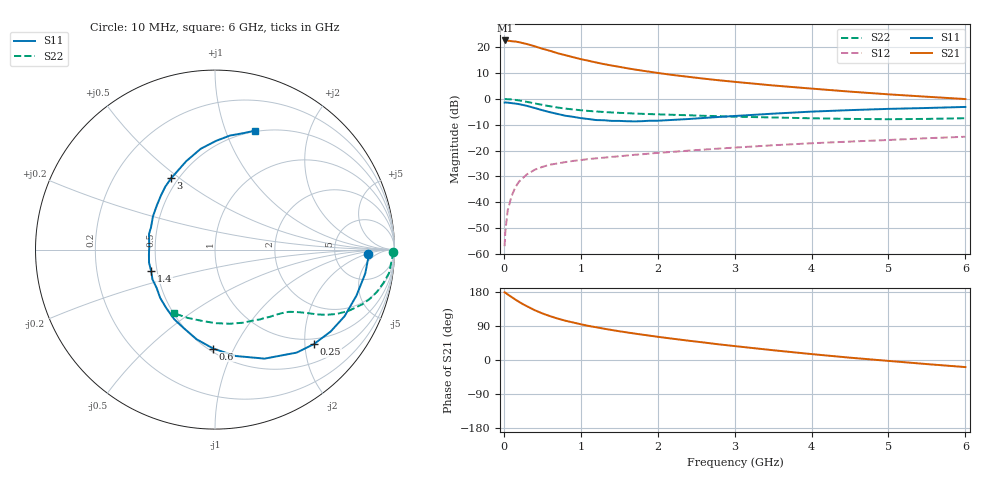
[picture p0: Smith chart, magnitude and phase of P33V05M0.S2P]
! SIEMENS Small Signal Semiconductors
! BFP181
! Si NPN RF Bipolar Junction Transistor in SOT143
! VCE = 3 V  IC = 5 mA
! Common Emitter S-Parameters:  March  1996
# GHz  S  MA  R  50
!  f  S11  S21  S12  S22
! GHz  MAG  ANG  MAG  ANG  MAG  ANG  MAG  ANG
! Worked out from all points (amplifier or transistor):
!   36 points, 10 MHz to 6 GHz, reference 50 ohm
!   highest |S21| = 22.7 dB at 20 MHz (marker M1)
!   |S21| within 3 dB of that: start of sweep to 478.8 MHz
!   unconditionally stable (mu >= 1): 1.667 GHz to end of sweep
!   at 250 MHz: K = 0.21, MSG = 26.1 dB, |S12| = -30.6 dB
!   at 1.4 GHz: K = 0.91, MSG = 17.7 dB, |S12| = -22.5 dB
!   at 6 GHz: K = 1.04, MAG = 6.0 dB, |S12| = -14.7 dB
!   lowest NFmin = 1.55 dB at 450 MHz
!   S11 on the Smith chart (normalised r, x): 10 MHz: 12, -2; 250 MHz: 0.88, -2.20; 600 MHz: 0.53, -0.83; 1.4 GHz: 0.46, -0.13; 3 GHz: 0.46, +0.47; 6 GHz: 0.49, +1.27
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0.01  0.8511 -1.8  13.5 178.6  0.0014 85.4  0.9902 -0.7
0.02  0.8542 -3.6  13.57 177.6  0.0027 85.9  0.9927 -1.5
0.05  0.8477 -9.0  13.47 173.1  0.0069 87.3  0.9851 -3.9
0.15  0.8117 -27.2  12.93 159.5  0.0195 74.8  0.9561 -11.3
0.2  0.7897 -35.3  12.54 153.1  0.0252 71.4  0.9325 -14.6
0.25  0.7621 -43.7  12.03 147.1  0.0295 67.5  0.9058 -17.6
0.3  0.7323 -51.6  11.57 141.9  0.0345 63.8  0.8764 -20.3
0.4  0.6675 -65.5  10.47 131.6  0.0423 57.6  0.8183 -24.7
0.5  0.6039 -79.0  9.387 123.0  0.0481 52.9  0.7663 -27.9
0.6  0.5518 -91.0  8.548 115.7  0.0531 49.3  0.7199 -30.3
0.7  0.5103 -101.5  7.672 109.3  0.0563 46.8  0.6804 -32.1
0.8  0.4715 -111.5  7.035 103.7  0.0596 44.9  0.6492 -33.4
0.9  0.4499 -120.2  6.436 99.0  0.0628 43.4  0.6242 -34.5
1.1  0.4072 -138.6  5.487 90.0  0.0682 41.4  0.5851 -36.6
1.4  0.375 -161.9  4.438 79.3  0.0752 39.7  0.5463 -39.4
1.8  0.3703 172.3  3.525 66.9  0.0846 38.5  0.5139 -43.5
2.2  0.3922 151.8  2.903 56.0  0.0943 37.3  0.4915 -48.4
3  0.4664 121.6  2.142 36.7  0.1139 33.9  0.4525 -60.1
3.5  0.5177 108.1  1.822 25.8  0.1263 31.3  0.4365 -68.9
4.5  0.6061 89.4  1.384 6.1  0.1489 24.9  0.4097 -89.8
5.5  0.6667 76.5  1.101 -10.8  0.173 19.4  0.4099 -111.9
6  0.6991 71.4  0.993 -18.7  0.1848 15.8  0.4222 -123.2
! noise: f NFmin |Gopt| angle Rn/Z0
0.45  1.55  0.48  17  0.36
0.9  1.65  0.4  35  0.34
1.8  2  0.18  88  0.34
